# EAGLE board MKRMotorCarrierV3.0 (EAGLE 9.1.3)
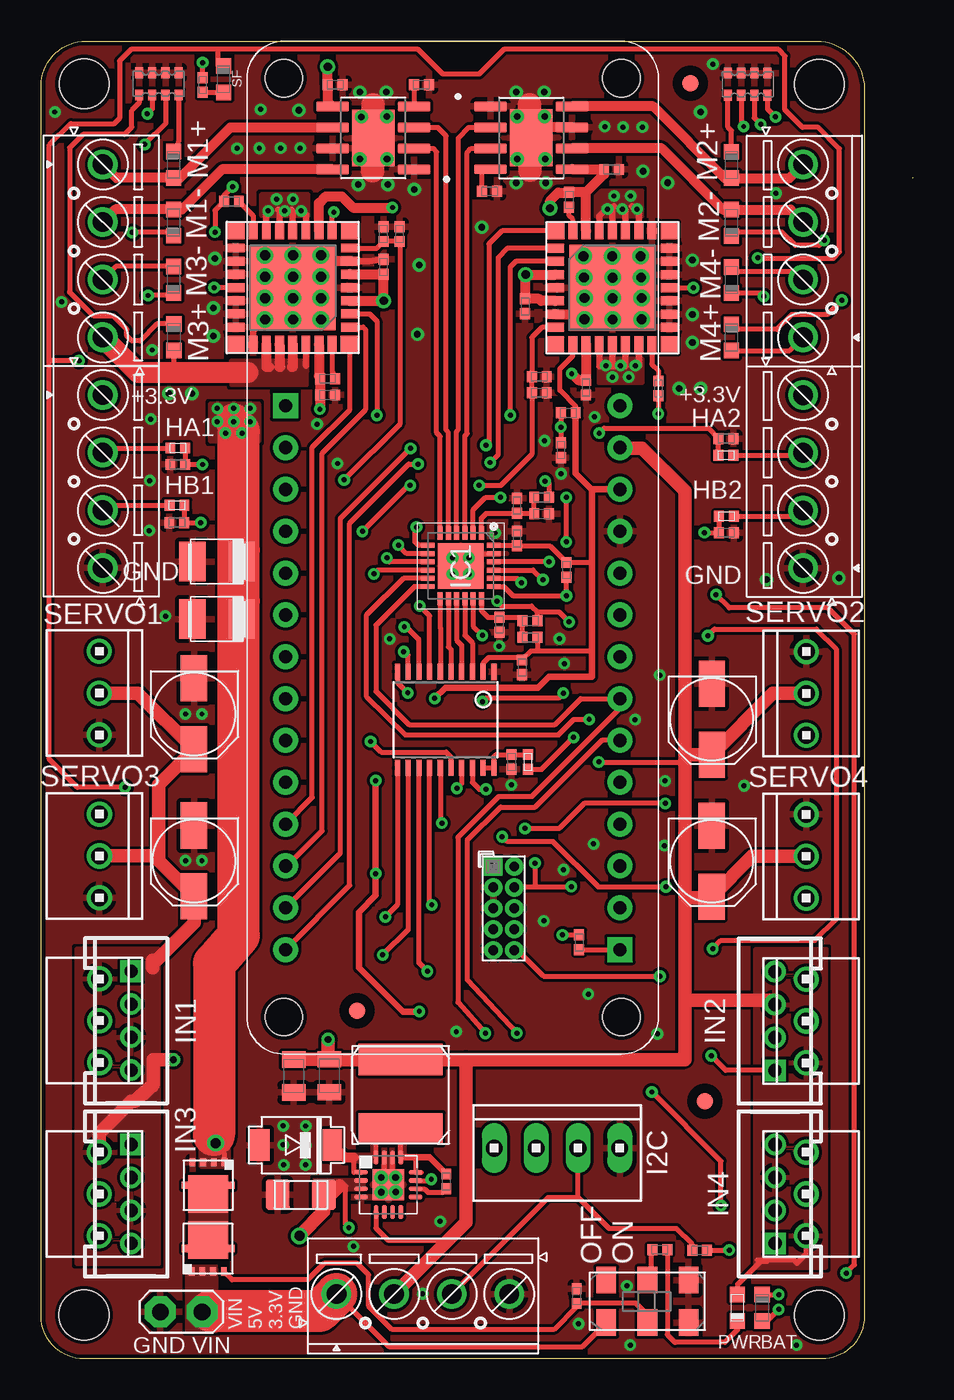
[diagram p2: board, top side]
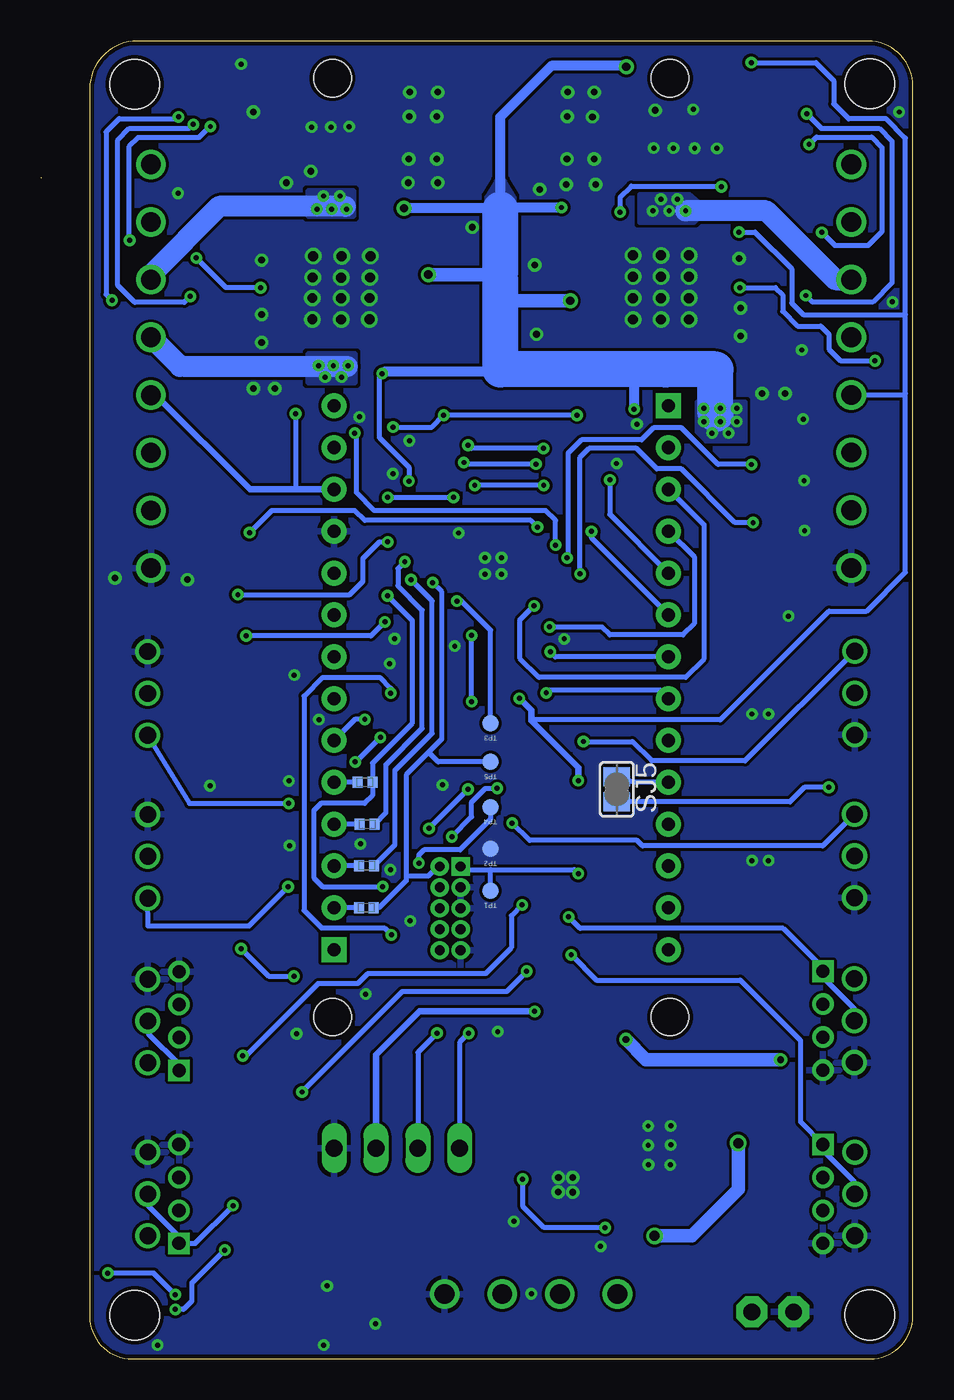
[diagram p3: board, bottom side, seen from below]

Size 52.95 x 80 mm. Coordinates in mm from the lower left corner, seen from the top.
Outline: 52.95,71.7 arc-90 52.95,71.7
Outline: 47.44,0 2.58,0 arc-90 0,2.58 0,77.28 arc-90 2.73,80 47.12,80 arc-90 50,77.12 50,2.56 arc-90 47.44,0
Copper layers (1*16): Top 0.035mm / dielectric 1.5mm / Bottom 0.035mm
Design rules "default *": minimum track width 0.3mm, minimum drill 0.3mm, track to track 7mil, track to pad 7mil, pad to pad 7mil, via to via 7mil, smd to smd 6mil, copper to edge 10mil, drill to drill 10mil, minimum pad ring 10mil, minimum via ring 8mil, stop-mask expansion 0.1mm, vias tented up to drill 0.5mm, thermal gap 10mil
Holes 3 mm at 2.6,2.66 47.26,2.64 47.27,77.39 2.61,77.41

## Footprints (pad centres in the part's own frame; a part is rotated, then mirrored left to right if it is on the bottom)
0402-1005X55N = smd 0.62 x 0.62: 1 -0.45,0; 2 0.45,0
SMC_B = smd 1.6 x 2.4: + -1.5,0; - 1.5,0
PANASONIC_C = smd 1.6 x 2.8: + 0,-2.15; - 0,2.15
C1206 = smd 1.8 x 1.45: 1 0,1.4; 2 0,-1.4
PINHEAD_2X05_127 = drill 0.6 pad 1.016 square: 1 -0.635,2.54 | drill 0.6 pad 1.016: 2 0.635,2.54; 3 -0.635,1.27; 4 0.635,1.27; 5 -0.635,0; 6 0.635,0; 7 -0.635,-1.27; 8 0.635,-1.27; 9 -0.635,-2.54; 10 0.635,-2.54
0805-R2013X50N = smd 0.95 x 1.45: 1 -1,0; 2 1,0
SOD-128 = smd 1.2 x 1.9: P$1 -2.2,0; P$2 2.2,0
LEDC1608X80N-AK = smd 0.9 x 0.95: A 0.8,0; C -0.8,0
QFN50P400X400X90-25N = smd 0.8 x 0.3: 1 -2,1.25; 2 -2,0.75; 3 -2,0.25; 4 -2,-0.25; 5 -2,-0.75; 6 -2,-1.25; 13 2,-1.25; 14 2,-0.75; 15 2,-0.25; 16 2,0.25; 17 2,0.75; 18 2,1.25 | smd 0.3 x 0.8: 7 -1.25,-2; 8 -0.75,-2; 9 -0.25,-2; 10 0.25,-2; 11 0.75,-2; 12 1.25,-2; 19 1.25,2; 20 0.75,2; 21 0.25,2; 22 -0.25,2; 23 -0.75,2; 24 -1.25,2 | smd 2.75 x 2.75: 25 0,0
MODULINO-3SM = drill 1.016: 1 2.54,0; 2 0,0; 3 -2.54,0
HW4-2.0 = drill 0.8 pad 1.27 square: 1 -3,0 | drill 0.8 pad 1.27: 2 -1,0; 3 1,0; 4 3,0
1X02 = drill 1.016 pad 1.88 octagon: 1 0,0; 2 2.54,0
6X6_NON-STANDARD = smd 1.9 x 5.1: P$1 -2.1,0; P$2 2.1,0
DFN3X3_8L = smd 0.5 x 0.35: P$1 -1.4,1.05; P$2 -1.4,0.4; P$3 -1.4,-0.25; P$4 -1.4,-0.9 | smd 2.28 x 2.45: P$5 0.51,0.055 | smd 0.43 x 0.38: P$6 0,1.47; P$7 0,-1.36
CAY16 = smd 0.5 x 0.65: 1 -1.2,-0.675; 2 -0.4,-0.675; 3 0.4,-0.675; 4 1.2,-0.675; 5 1.2,0.675; 6 0.4,0.675; 7 -0.4,0.675; 8 -1.2,0.675
SJ = smd 1.168 x 1.6: 1 -0.762,0; 2 0.762,0
TP-1.00MM = smd 1 x 1 bottom: X 0,0
MODULINO-4 = drill 1.016 long: 1 5.08,0; 2 2.54,0; 3 0,0; 4 -2.54,0
TSSOP20 = smd 0.305 x 0.991: 1 -2.925,-2.918; 2 -2.275,-2.918; 3 -1.625,-2.918; 4 -0.975,-2.918; 5 -0.325,-2.918; 6 0.325,-2.918; 7 0.975,-2.918; 8 1.625,-2.918; 9 2.275,-2.918; 10 2.925,-2.918; 11 2.925,2.918; 12 2.275,2.918; 13 1.625,2.918; 14 0.975,2.918; 15 0.325,2.918; 16 -0.325,2.918; 17 -0.975,2.918; 18 -1.625,2.918; 19 -2.275,2.918; 20 -2.925,2.918
QFN16 = smd 0.85 x 0.3: 1 -1.655,0.75; 2 -1.655,0.25; 3 -1.655,-0.25; 4 -1.655,-0.75; 9 1.655,-0.75; 10 1.655,-0.25; 11 1.655,0.25; 12 1.655,0.75 | smd 0.3 x 0.85: 5 -0.75,-1.655; 6 -0.25,-1.655; 7 0.25,-1.655; 8 0.75,-1.655; 13 0.75,1.655; 14 0.25,1.655; 15 -0.25,1.655; 16 -0.75,1.655 | smd 1.905 x 1.905: 17 0,0
32-PQFN(8X8) = smd 1.05 x 1.05: 1 -3.44,3.46; 9 -3.46,-3.46; 17 3.46,-3.46; 25 3.46,3.46 | smd 1.05 x 0.54: 2 -3.46,2.4; 3 -3.46,1.6; 4 -3.46,0.8; 5 -3.46,0; 6 -3.46,-0.8; 7 -3.46,-1.6; 8 -3.46,-2.4; 18 3.46,-2.4; 19 3.46,-1.6; 20 3.46,-0.8; 21 3.46,0; 22 3.46,0.8; 23 3.46,1.6; 24 3.46,2.4 | smd 0.54 x 1.05: 10 -2.4,-3.46; 11 -1.6,-3.46; 12 -0.8,-3.46; 13 0,-3.46; 14 0.8,-3.46; 15 1.6,-3.46; 16 2.4,-3.46; 26 2.4,3.46; 27 1.6,3.46; 28 0.8,3.46; 29 0,3.46; 30 -0.8,3.46; 31 -1.6,3.46; 32 -2.4,3.46 | smd 5.2 x 5.2: EPAD 0,0
SOIC127P600X170-8N = smd 1.97 x 0.6: 1 -2.475,1.905; 2 -2.475,0.635; 3 -2.475,-0.635; 4 -2.475,-1.905; 5 2.475,-1.905; 6 2.475,-0.635; 7 2.475,0.635; 8 2.475,1.905 | smd 2.58 x 3.45: 9 0,0
MKRBOARD-4CARRIER = drill 0.8 pad 1.524: 0 42.455,2.34; 1 44.995,2.34; 2 47.535,2.34; 3 50.075,2.34; 4 52.615,2.34; 5 55.155,2.34; 5V 22.135,22.66; 7 52.615,22.66; 8 50.075,22.66; 9 47.535,22.66; 10 44.995,22.66; 11 42.455,22.66; 12 39.915,22.66; 13 37.375,22.66; 14 34.835,22.66; A0 24.675,2.34; A1 27.215,2.34; A2 29.755,2.34; A3 32.295,2.34; A4 34.835,2.34; A5 37.375,2.34; A6 39.915,2.34; GND 29.755,22.66; RST 32.295,22.66; VCC 27.215,22.66; VIN 24.675,22.66 | drill 0.8 pad 1.524 square: 6 55.155,22.66; AREF 22.135,2.34 | hole 2.25: 59.25,2.25; 59.25,22.75; 2.25,22.75; 2.25,2.25
FD-1-1.5 = smd 1.016 x 1.016: P$1 0,0
CL-SB-22A = smd 1.2 x 1.6: P$1 -2.5,-1.29; P$2 0,-1.29; P$3 2.5,-1.29; P$4 -2.5,1.29; P$5 0,1.29; P$6 2.5,1.29
OSTTE/4 = drill 1.2: 1 -5.25,0; 2 -1.75,0; 3 1.75,0; 4 5.25,0

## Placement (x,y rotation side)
C1  100n  [0402-1005X55N]  28.9,49.81 90 top
C2  47uF  [SMC_B]  10.68,48.4 180 top
C3  47uF  [SMC_B]  10.68,44.91 180 top
C4  47n  [0402-1005X55N]  32.07,70.37 270 top
C5  150uF  [PANASONIC_C]  9.28,30.23 0 top
C6  47n  [0402-1005X55N]  17.4,59.51 0 top
C7  100n  [0402-1005X55N]  17.4,58.52 0 top
C8  100n  [0402-1005X55N]  34.65,72.21 0 top
C9  100n  [0402-1005X55N]  33.1,58.97 270 top
C10  1u  [0402-1005X55N]  21.77,68.29 270 top
C11  1u  [0402-1005X55N]  30.26,58.66 180 top
C12  100n  [0402-1005X55N]  29.4,63.9 270 top
C13  150uF  [PANASONIC_C]  40.73,30.21 0 top
C14  10n  [0402-1005X55N]  41.6,55.87 180 top
C15  10n  [0402-1005X55N]  41.62,50.15 0 top
C16  10n  [0402-1005X55N]  8.24,50.77 0 top
C17  10n  [0402-1005X55N]  8.3,54.3 180 top
C18  100n  [0402-1005X55N]  20.8,66.3 90 top
C19  100n  [0402-1005X55N]  28.58,36.24 270 top
C20  100n  [0402-1005X55N]  29.22,41.98 90 top
C21  100n  [0402-1005X55N]  28.9,51.8 90 top
C22  100n  [0402-1005X55N]  27.84,44.57 270 top
C23  10n  [0402-1005X55N]  32.53,3.81 270 top
C25  150uF  [PANASONIC_C]  9.28,39.16 0 top
C26  100n  [0402-1005X55N]  17.86,77.35 0 top
C31  150uF  [PANASONIC_C]  40.74,38.83 0 top
CBST  100n  [0402-1005X55N]  24.61,10.77 90 top
CBYPASS  10uF  [C1206]  15.77,9.97 90 top
CN1  DNP  [PINHEAD_2X05_127]  28.1,27.35 0 top
COUT1  22u  [0805-R2013X50N]  17.5,17.19 90 top
COUT2  22u  [0805-R2013X50N]  15.34,17.17 270 top
D1  40V/5A  [SOD-128]  15.49,12.98 180 top
DL1  YELLOW  [LEDC1608X80N-AK]  8.05,72.5 270 top
DL2  YELLOW  [LEDC1608X80N-AK]  8.05,68.99 90 top
DL3  YELLOW  [LEDC1608X80N-AK]  8.05,65.52 90 top
DL4  YELLOW  [LEDC1608X80N-AK]  8.06,62.03 270 top
DL5  YELLOW  [LEDC1608X80N-AK]  41.93,62.01 270 top
DL6  YELLOW  [LEDC1608X80N-AK]  41.93,65.5 90 top
DL7  YELLOW  [LEDC1608X80N-AK]  41.93,68.98 90 top
DL8  YELLOW  [LEDC1608X80N-AK]  41.93,72.49 270 top
DL9  ORANGE  [LEDC1608X80N-AK]  11.09,77.69 270 top
DL10  ORANGE  [LEDC1608X80N-AK]  43.8,3.1 270 top
FRAME1  DNP  [FRAME-NO-BAN]  not placed on the board
FRAME2  DNP  [FRAME]  not placed on the board
IC1  ATSAMD11D14A-MNT  [QFN50P400X400X90-25N]  25.49,48.14 270 top
IN1  DNP  [MODULINO-3SM]  3.55,20.53 90 top
IN2  DNP  [MODULINO-3SM]  46.47,20.51 270 top
IN3  DNP  [MODULINO-3SM]  3.53,10.01 90 top
IN4  DNP  [MODULINO-3SM]  46.47,10.01 270 top
J1  DNP  [HW4-2.0]  5.46,10.01 270 top
J2  DNP  [HW4-2.0]  5.46,20.53 270 top
J3  DNP  [HW4-2.0]  44.58,10.01 90 top
J4  DNP  [HW4-2.0]  44.57,20.51 90 top
JP2  M02PTH  [1X02]  7.24,2.85 0 top
LOUT  4.7uH/4A/35mO  [6X6_NON-STANDARD]  21.84,16.07 90 top
ON  GREEN  [LEDC1608X80N-AK]  42.3,3.1 90 top
Q1  AON7407  [DFN3X3_8L]  10.09,10.53 270 top
Q3  AON7407  [DFN3X3_8L]  10.2,6.7 90 top
R1  330R  [0402-1005X55N]  37.58,6.62 180 top
R2  39R  [0402-1005X55N]  29.7,44.8 0 top
R3  10k  [0402-1005X55N]  30.4,52.3 0 top
R4  140R  [0402-1005X55N]  41.6,54.86 0 top
R5  140R  [0402-1005X55N]  41.63,51.15 0 top
R6  140R  [0402-1005X55N]  8.25,51.83 180 top
R7  140R  [0402-1005X55N]  8.3,55.3 180 top
R8  DNP  [0402-1005X55N]  33.28,35 180 bottom
R9  3k3  [0402-1005X55N]  30.4,51.3 180 top
R10  200K  [0402-1005X55N]  29.57,36.24 270 top
R11  1k  [0402-1005X55N]  9.81,77.34 270 top
R12  10k  [0402-1005X55N]  32.02,57.43 0 top
R13  DNP  [0402-1005X55N]  33.15,32.46 180 bottom
R14  22K  [0402-1005X55N]  27.24,70.89 180 top
R15  DNP  [0402-1005X55N]  33.18,29.93 180 bottom
R16  DNP  [0402-1005X55N]  33.2,27.39 180 bottom
R17  22K  [0402-1005X55N]  23.1,77.35 180 top
R18  DNP  [0402-1005X55N]  31.57,55.17 90 top
R19  1k  [0402-1005X55N]  37.49,58.92 90 top
R20  1k  [0402-1005X55N]  11.56,70.27 0 top
R21  0R  [0402-1005X55N]  32.68,25.29 90 top
R22  270R  [0402-1005X55N]  30.26,59.62 180 top
R23  270R  [0402-1005X55N]  20.79,68.29 270 top
R24  330R  [0402-1005X55N]  40,6.6 0 top
R25  1k  [0402-1005X55N]  31.91,47.9 270 top
R26  10k  [0402-1005X55N]  29.7,43.8 180 top
RN2  1k  [CAY16]  42.92,77.39 180 top
RN4  1k  [CAY16]  7.15,77.41 180 top
SERVO1  DNP  [MODULINO-3SM]  3.53,40.42 90 top
SERVO2  DNP  [MODULINO-3SM]  46.48,40.4 270 top
SERVO3  DNP  [MODULINO-3SM]  3.54,30.53 90 top
SERVO4  DNP  [MODULINO-3SM]  46.47,30.51 270 top
SJ5  [SJ]  17.98,34.58 270 bottom
TP1  DNP  [TP-1.00MM]  25.64,28.42 180 top
TP2  DNP  [TP-1.00MM]  25.64,30.96 180 top
TP3  DNP  [TP-1.00MM]  25.64,38.58 180 top
TP4  DNP  [TP-1.00MM]  25.64,33.5 180 top
TP5  DNP  [TP-1.00MM]  25.64,36.24 180 top
TWI  -  [MODULINO-4]  32.61,12.79 180 top
U1  LSF0108  [TSSOP20]  24.57,38.8 180 top
U2  TS30013  [QFN16]  21.09,10.57 0 top
U3  MC33926PNB  [32-PQFN(8X8)]  15.28,65.04 180 top
U4  DRV8871  [SOIC127P600X170-8N]  20.18,74.12 180 top
U5  MC33926PNB  [32-PQFN(8X8)]  34.7,65.03 0 top
U7  DRV8871  [SOIC127P600X170-8N]  29.77,74.13 0 top
U$1  MKRBOARD4CARRIER  [MKRBOARD-4CARRIER]  12.5,80 270 top
U$33  DNP  [FD-1-1.5]  19.18,21.14 0 top
U$34  DNP  [FD-1-1.5]  40.32,15.63 0 top
U$35  DNP  [FD-1-1.5]  39.42,77.44 0 top
U$38  CL-SB-22A-02T  [CL-SB-22A]  36.83,3.49 180 top
X1  OSTTE/4  [OSTTE/4]  46.28,67.27 90 top
X2  OSTTE/4  [OSTTE/4]  46.28,53.26 90 top
X3  OSTTE/4  [OSTTE/4]  3.74,53.27 270 top
X6  OSTTE/4  [OSTTE/4]  3.74,67.27 270 top
X8  OSTTE/4  [OSTTE/4]  23.19,3.93 0 top

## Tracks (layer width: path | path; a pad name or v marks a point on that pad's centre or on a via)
+3.3V  (via drill 0.3)
  Top 0.305: U5.10 | U$1.VCC 35.15,52.8 | R11.1 v9.81,78.7 | R19.1 v37.49,57.38 | 30.1,42.99 29.78,42.99 C20.2 29.07,42.58 27.18,42.58 26.84,42.24 U1.2 | 30.1,42.99 33.47,42.99 | 32.61,9.8 TWI.3 | IC1.24 28.92,49.39 C1.1 30.91,49.36 R25.1 33.42,48.35 33.47,48.4 | U3.10 17.68,69.52 v17.78,69.62 | 32.61,9.8 34.51,7.9 38.6,7.9 39.55,6.95 R24.1 | X8.3 30.81,9.8 32.61,9.8 | 32.3,61.1 U5.10 | v10.56,68.41 10.56,69.72 R20.1 11.11,70.64 v11.63,71.16 | U5.10 32.3,60.9 31.5,60.1 31.5,58.8 32.47,57.83 R12.2 | R26.1 30.15,43.04 30.1,42.99
  Top 0.406: U$1.VCC 33.49,52.78 33.47,52.77 | v22.97,21.09 v22.96,21.08 21.97,21.08 19.3,23.75 19.3,27.12 20.32,28.14 v20.32,29.46 v20.32,35.11 | 33.47,52.77 33.47,48.4 33.47,42.99 33.47,41.4 30.84,41.4 30.19,40.75 24.55,40.75 v23.9,40.1 | R12.2 32.47,53.77 33.47,52.77
  Bottom 0.305: v9.81,78.7 5.89,78.7 4.8,77.61 4.8,76.19 3.89,75.28 1.61,75.28 0.45,74.12 0.45,63.4 | 0.45,58.6 0.45,47.75 2.8,45.4 5.1,45.4 11.7,38.8 23.1,38.8 23.16,38.73 | 0.45,58.6 0.45,63.4 | v37.49,57.38 37.49,52.78 | v17.78,69.62 17.78,70.52 17.1,71.2 11.67,71.2 v11.63,71.16 | 25.64,29.7 27.38,29.7 CN1.1 | 25.64,29.7 20.56,29.7 v20.32,29.46 | 0.45,63.4 6.66,63.4 7.35,64.09 7.35,66.17 9.59,68.41 v10.56,68.41 | TP1.X 25.64,29.7 | X3.1 0.53,58.52 0.45,58.6
  Bottom 0.406: U$1.VCC 37.49,52.78 40.26,52.78 45.98,58.51 X2.4 | v22.97,21.09 29.98,21.09 32.61,18.46 TWI.3 | v20.32,35.11 20.32,35.89 23.16,38.73 23.16,39.37 v23.9,40.1
+5V  (via drill 0.3, 0.4)
  Top 0.305: U2.5 20.34,7.93 21.07,7.2 24.71,7.2 25,7.5 | v33.87,36.24 33.89,36.22 39.07,36.22 39.1,36.25 | v32.34,37.73 30.4,35.79 R10.2 | IN4.1 46.47,6.37 45.9,5.8 45.7,6 43.5,6 43.6,5.9 44.1,5.9 44,6 43.8,6 42.3,4.5 ON.A
  Top 0.406: 39.11,18.18 39.1,18.17
  Top 0.813: LOUT.P$2 | LOUT.P$2 17.43,18.17 | 15.27,18.17 COUT2.1 15.36,18.19 COUT1.2 17.43,18.17 | LOUT.P$2 25.8,18.17 | 25.8,18.17 39.1,18.17 39.1,21.76 | 39.1,21.76 39.1,27.99 | 39.1,27.99 39.1,36.25 39.1,36.61 | 39.1,36.61 39.1,52.7 36.5,55.3 35.19,55.3 U$1.VIN | 39.1,36.61 39.17,36.68 C31.+ 44.46,40.4 SERVO2.2 | IN3.1 3.53,13.71 5.46,15.64 5.69,15.64 6.8,16.65 6.8,18.16 v8.04,18.16 | 6.77,24.21 6.77,23.96 | 6.77,23.96 6.77,23.73 | J4.3 44.52,21.76 39.1,21.76 | 39.1,27.99 40.66,27.99 C13.+ 43.18,30.51 SERVO4.2 | 7.13,30.23 C5.+ 9.28,26.47 6.77,23.96 | 7.13,30.23 7.13,34.86 C25.+ 5.87,40.42 SERVO1.2 | SERVO3.2 6.83,30.53 7.13,30.23 | 17.43,18.17 v17.43,19.39 | 25.8,18.17 25.8,8.29 25,7.5 X8.2
  Bottom 0.305: v33.87,36.24 33.83,36.24 v32.34,37.73
  Bottom 0.813: v8.04,18.16 16.2,18.16 v17.43,19.39
  pour Top: 7.13,24.88 2.16,24.88 2.16,5.8 7.14,5.8
  pour Top: 43.4,24.85 43.4,5.57 47.68,5.57 47.68,24.12 47.7,24.85
+VM  (via drill 0.3, 0.5, 0.5 pad 0.25, 0.6)
  Top 0.305: U4.5 | U3.31 16.93,61.58 | Q1.P$1 11.14,12.46 v10.6,13.1 | U2.11 23.62,10.82 v23.7,10.9 | R3.2 30.85,53.15 30.71,53.29 v30.61,53.29 | C2.+ 12.2,48.42 12,49.1 | C3.+ 12.2,44.93 12,46 | v18.69,7.96 18.5,8.15 18.5,10.5
  Top 0.61: U5.11 C9.1 32.63,59.42 v32.23,59.82 | U3.11 16.88,70.17 17.28,70.57 18.26,70.57 18.94,69.89 v21.33,69.89 v21.34,69.9 | v16.93,57.66 16.95,57.96 C7.1 C6.1 16.88,59.68 U3.31 | U5.31 33.1,70.82 | 33.1,70.82 C4.1 32.05,70.8 31.4,70.8 30.91,70.31 v30.91,69.86 | U7.5 34.2,72.22 C8.1 34.2,71.92 33.1,70.82 | U5.4 v29.43,65.83 29.4,65.8 C12.1 30.25,64.35 30.37,64.23 U5.6 | U3.4 v20.81,64.24 v20.8,64.25 C18.1 U3.6 | U4.5 17.41,76.32 C26.1 v17.41,78.45
  Top 0.813: CBYPASS.2 17.35,9.71 18.14,10.5 | 17.09,9.89 CBYPASS.2 | v15.69,7.47 17.17,8.95 CBYPASS.2
  Top 1.27: 10.5,13.6 10.5,13.2 v10.6,13.1
  Top 2.184: 12,56.3 v11.7,56.9
  Top 2.54: 12,56.3 12,49.1 12,46 12,25.7 10.5,24 10.5,13.6
  Bottom 0.305: v18.69,7.96 22.4,7.96 23.67,9.23 23.67,10.87 v23.7,10.9 | 25.27,59.92 25.06,59.92 25.06,60.07 | v30.61,53.29 30.61,54.14 32.4,55.93 32.4,59.65 v32.23,59.82
  Bottom 0.61: 25.06,69.78 25.06,69.86 | 25.06,69.86 v30.91,69.86 | v21.34,69.9 25.06,69.9 | 25.06,69.9 25.06,69.86 | 15,60.07 16.93,59.97 16.95,59.95 16.93,59.93 v16.93,57.66 | 25.27,59.92 32.13,59.92 v32.23,59.82 | 25.06,69.9 25.06,75.4 21.96,78.5 17.46,78.5 v17.41,78.45
  Bottom 0.813: v10.6,13.1 10.6,10.3 13.43,7.47 v15.69,7.47 | 24.9,65.84 25.06,66 | v29.43,65.83 25.39,65.83 25.06,65.5 | v20.81,64.24 25.06,64.24
  Bottom 1.27: 25.06,64.14 25.06,64.24
  Bottom 1.778: 25.06,65.5 25.06,66 | 25.06,64.1 25.06,64.24 25.06,64.4
  Bottom 2.184: 25.06,64.4 25.06,65.5 | 25.06,66 25.06,69.78 | 11.98,57.35 11.98,60.07 15,60.07 25.06,60.07 25.06,64.1
  other vias: 10.7,57.7 11.7,57.7 12.7,57.7 10.7,56.9 12.7,56.9 11.2,56.2 12.2,56.2
  pour Top (no thermals): 9.7,11.7 11.4,11.7 11.4,13.4 9.7,13.4
  pour Top: 13.2,55.7 10.3,55.7 10.3,58 13.2,58
  pour Bottom: 13.1,58.1 10.2,58.1 10.2,55.7 13.1,55.7
  pour Bottom: 24.2,69.9 24.2,70.5 24.8,71.5 25.3,71.5 25.9,70.5 25.9,69.9
  pour Top (no thermals): 19.61,10.85 16.57,10.85 17.8,10.3 19.6,10.3
/SF  (via drill 0.3)
  Top 0.305: U3.21 v10.51,65.04 | U5.21 v39.62,65.03 | DL9.C 10.75,78.53 10.75,79.5 | 10.75,79.5 5.46,79.5 4.76,78.8 4.76,75.32 4.44,75 1.8,75 0.5,73.7 0.5,60.6 | v5.1,34.7 2.2,34.7 0.5,36.4 0.5,60.6 | v2.3,60.6 0.5,60.6 | v43.53,66.84 43.47,66.8 48.1,66.8 48.5,67.2 48.5,73.47 47.2,74.77 46.25,74.77 45.19,75.83 45.19,79.11 44.8,79.5 28.1,79.5 26.6,78 24.4,78 22.9,79.5 10.75,79.5
  Bottom 0.305: SJ5.2 7.46,33.82 6.58,34.7 v5.1,34.7 | v39.62,65.03 41.72,65.03 v43.53,66.84 | v10.51,65.04 8.34,65.04 7.9,64.6 7.9,63.6 7,62.7 5.6,62.7 5.1,62.2 5.1,61.3 4.4,60.6 v2.3,60.6
A1  (via drill 0.3)
  Top 0.305: U1.7 23.59,45.12 v23,45.71
  Bottom 0.305: U$1.A1 12.67,50.62 12.67,42.51 13.81,41.37 22.7,41.37 23.88,42.55 23.88,44.83 v23,45.71
A2  (via drill 0.3)
  Top 0.305: U1.8 22.95,43.66 22.16,44.44 v22.06,44.44
  Bottom 0.305: U$1.A2 13.28,48.69 13.28,44.63 13.96,43.95 18.4,43.95 18.88,44.43 v22.05,44.43 v22.06,44.44
A5  (via drill 0.3)
  Top 0.305: U1.9 22.3,42.73 22.09,42.93 v22.02,42.93
  Bottom 0.305: 21.85,42.83 21.95,42.93 v22.02,42.93 21.71,42.62 U$1.A5
A6  (via drill 0.3)
  Top 0.305: U1.10 21.64,41.05 v22.27,40.43
  Bottom 0.305: U$1.A6 15.36,40.6 22.1,40.6 v22.27,40.43
FB_M3  (via drill 0.3)
  Top 0.305: v18.4,53.36 21.79,56.75 21.79,67.82 C10.2 R23.2 20.39,67.44 U3.8
  Bottom 0.305: v18.4,53.36 18.4,51.27 U$1.A3
FB_M4  (via drill 0.3)
  Top 0.305: v19.52,50.24 22.31,53.03 v22.42,53.03 | v26.61,53.03 27.93,53.03 29.81,54.91 C11.2 R22.2 29.81,62.01 30.43,62.63 U5.8
  Bottom 0.305: v22.42,53.03 v26.61,53.03 | U$1.A4 19.52,49.84 v19.52,50.24
GND  (via drill 0.3, 0.4, 0.41, 0.6)
  Top 0.305: U2.15 20.84,11.18 v20.66,11.01 | 21.33,12.2 21.33,11.21 v21.53,11.01 v21.52,11.01 | 25.09,48.95 IC1.25 25.79,48.14 26.54,48.89 IC1.23 | 33.14,64.33 33.13,64.33 v33.01,64.41 | 29.52,74.78 29.52,74.38 U7.9 | v32.98,65.65 34.71,65.05 v34.72,65.64 36.34,65.04 v36.45,65.65 | 33.14,63.03 33.13,63.03 v33.01,63.11
  Top 0.406: U3.7 19.89,66.64 C18.2 | U3.26 12.88,62.38 v13.6,63.1
  Top 0.61: U7.7 29.52,74.78 v28.92,75.43 | 33.14,64.33 33.18,64.29 33.18,64.41 U5.EPAD | 17.3,66.94 v17,67 17.36,66.64 U3.7 | U5.7 32.93,63.43 33,63.5 v33,64.4 v33.01,64.41 | 33.14,63.03 33.18,62.99 33.18,63.11 34.7,63.73 | v33,63.1 v33.01,63.11
  Top 1.422: 29.68,72.46 29.68,72.15 | 29.67,76.15 29.67,75.84 | 20.13,72.45 20.13,72.14 | 20.17,76.15 20.17,75.84
  other vias: 20.66,10.12 21.54,10.12 19.46,75.41 21.01,72.85 20.99,75.42 7.55,45.09 16.07,11.79 25.21,19.87 18.96,6.83 14.73,11.78 14.71,14.14 16.07,14.13 35.78,0.83 23.18,3.95 19.36,72.85 35.59,4.43 6.58,50.28 6.61,53.32 30.58,75.42 28.92,72.84 30.62,72.84 14.71,12.98 32.65,2.13 6.66,57.05 32.95,66.95 34.69,66.94 34.72,64.4 36.48,64.41 36.42,66.95 17,64.4 15.3,65.7 13.6,67 13.6,65.7 13.6,64.4 15.3,64.4 15.3,67 17,65.7 44.64,70.77 1.24,64.17 30.59,55.74 33.62,57.19 28.57,34.85 13.34,75.86 0.83,75.7 6.75,61.25 40.8,78.61 25.98,47.64 14.54,73.51 13.26,73.5 11.9,73.49 15.73,73.51 33.23,22.14 37.9,35.09 16.07,12.96 31.77,42.21 37.85,31.16 30.54,26.59 31.48,43.72 34.23,74.81 35.34,74.78 36.52,74.78 18,54.36 31.59,53.74 24.23,8.34 27.59,50.14 42.7,34.79 15.3,63.1 17,63.1 34.72,63.1 36.48,63.11 28.86,76.91 30.56,76.91 30.66,71.41 19.36,76.91 20.96,76.91 28.86,71.41 15.66,75.81 40.06,75.7 36.56,72.11 19.26,71.31 21.06,71.31 22.96,66.41 22.86,62.2 22.66,71 10.46,62.1 10.46,63.8 9.16,58.6 10.56,66.81 39.56,63.41 39.56,66.7 38.06,71.41 7.76,58.6 38.76,58.91 40.06,58.91 39.56,61.7 26.76,68.7 45.88,0.83 24.98,48.64 25.98,48.64 24.98,47.64 48.46,47.41 44.06,47.3 16.76,56.75 8.77,30.25 9.77,30.25 8.77,39.15 9.77,39.15 31.73,29.69 36.08,38.81 33.55,31.26 21.18,43.71 37.58,41.51 37.44,19.74 27.82,43.27
  pour Top (rank 6): 49.95,79.95 0.46,80.05 arc90 0.2,79.79 -0.13,-1.77 49.92,-1.77
  pour Bottom (rank 6): 0.05,79.8 -0.15,-1.79 48.01,-1.67 arc90 50.01,0.34 49.96,79.93
HA_E1  (via drill 0.3)
  Top 0.305: IC1.9 21.16,48.39 21,48.55 v21,48.63 | R7.1 C17.1 v9.8,54.3
  Bottom 0.305: v21,48.63 20.92,48.71 20.92,55 20.13,55.79 16.48,55.79 15.75,56.52 14.05,56.52 11.83,54.3 v9.8,54.3
HA_E2  (via drill 0.3)
  Top 0.305: R4.1 C14.2 40.52,56.5 34.2,56.5 v33.9,56.2 | IC1.8 22.21,48.89 v21.7,49.4
  Bottom 0.305: v21.7,49.4 21.7,50.9 22.3,51.5 32.7,51.5 33.8,52.6 33.8,56.1 v33.9,56.2
HB_E1  (via drill 0.3)
  Top 0.305: R6.1 C16.2 v9.7,50.77 | IC1.10 20.44,47.89 v20.21,47.66
  Bottom 0.305: v9.7,50.77 10.8,50.77 14.07,54.04 15.55,54.04 16.78,55.27 19.67,55.27 20.21,54.73 v20.21,47.66
HB_E2  (via drill 0.3)
  Top 0.305: R5.1 C15.1 v40.29,50.16 | IC1.7 22.91,49.39 22.7,49.6 22.7,50.4 v22.8,50.5
  Bottom 0.305: v22.8,50.5 23.2,50.9 33.3,50.9 33.9,51.5 38.95,51.5 v40.29,50.16
IN1_A6  (via drill 0.3)
  Top 0.305: U1.11 21.64,27.57 v20.91,26.83
  Bottom 0.305: IN1.2 3.55,21.25 5.46,23.16 J2.1 5.46,23.73 7.87,26.14 20.22,26.14 v20.91,26.83
IN1_M1
  Top 0.305: U4.3 24.09,74.75 24.6,74.25 24.6,56.39 24.74,56.25 IC1.5
IN1_M2
  Top 0.305: IC1.3 25.74,56.04 25.87,56.17 25.87,73.24 26.12,73.49 U7.3
IN1_M3
  Top 0.305: U3.2 19.56,62.64 19.7,62.5 19.7,57.61 17.07,54.98 17.07,32.05 14.94,29.93 U$1.3
IN1_M4  (via drill 0.3)
  Top 0.305: U5.2 28.34,67.43 27.77,66.86 27.77,54.92 v27.27,54.42 | U$1.5 18.74,28.75 18.74,50.73 22.33,54.32 v22.89,54.32
  Bottom 0.305: v22.89,54.32 27.17,54.32 v27.27,54.42
IN2_A1  (via drill 0.3)
  Top 0.305: U1.14 23.59,27.7 v23.73,27.56 | J4.1 41.59,17.51 v40.7,18.4
  Bottom 0.305: v23.73,27.56 24.38,26.91 24.38,24.97 25.96,23.39 33.11,23.39 33.7,22.8 36.1,22.8 40.5,18.4 v40.7,18.4 | IN2.2 46.47,19.77 44.57,17.87 J4.1
IN2_M1
  Top 0.305: IC1.6 24.24,56.01 24.03,56.22 24.03,73.27 23.82,73.48 U4.2
IN2_M2
  Top 0.305: IC1.4 25.24,56.32 25.34,56.42 25.34,74.12 25.99,74.77 U7.2
IN2_M3
  Top 0.305: U3.1 18.72,57.6 16.47,55.36 16.47,34.09 14.86,32.47 U$1.2
IN2_M4  (via drill 0.3)
  Top 0.305: U5.1 28,68.49 27.2,67.69 27.2,55.65 v27.02,55.47 v27.03,55.48 | v22.44,55.28 18.18,51.02 18.18,30.73 U$1.4
  Bottom 0.305: v22.44,55.28 26.83,55.28 v27.02,55.47
IN3_A5  (via drill 0.3)
  Top 0.305: U1.12 22.3,26.07 v20.75,24.52
  Bottom 0.305: v20.75,24.52 19.22,22.99 10.48,22.99 6.83,19.34 6.83,14.38 J1.1 5.46,12.65 3.53,10.72 IN3.2
IN4_A2  (via drill 0.3)
  Top 0.305: 22.96,35.87 U1.13 22.95,24.05 v23.46,23.53 | v41.3,9.3 41.3,12 v37.1,16.2
  Bottom 0.305: 31,22.31 30.99,22.31 | IN4.2 46.47,9.31 44.58,7.42 J3.1 43.59,7.01 v41.3,9.3 | v23.46,23.53 23.46,23.51 24.66,22.31 30.5,22.31 30.99,22.31 | v37.1,16.2 30.99,22.31
LED_S  (via drill 0.3)
  Top 0.305: IC1.2 26.24,51.54 27,52.3 v27.9,52.3 | DL10.C v44.8,3.9 | v41,46.4 41.8,45.6 47.8,45.6 49.4,44 49.4,5.7 v48.9,5.2 | v31.9,49.6 v31.9,52.3
  Bottom 0.305: v41,46.4 34.2,46.4 33.4,47.2 33.4,48.6 32.4,49.6 v31.9,49.6 | v31.9,52.3 v27.9,52.3 | v44.8,3.9 46.1,5.2 v48.9,5.2
M1+
  Top 0.61: U4.6 11.48,74.75 8.43,71.7 DL1.A 4.56,71.7 X6.1
M1-
  Top 0.61: U4.8 10.98,72.22 8.56,69.79 DL2.A 4.51,69.79 X6.2
M2+
  Top 0.61: U7.8 37.19,76.03 41.53,71.69 DL8.A 45.45,71.69 X1.4
M2-
  Top 0.61: U7.6 37.7,73.5 41.42,69.78 DL7.A 45.52,69.78 X1.3
M3+
  Top 0.305: DL4.A 8.06,59.91 8.04,59.89
  Top 0.406: U3.30 16.08,60.3
  Top 0.61: U3.29 15.28,60.22 15.23,60.22 | U3.28 14.48,60.22 14.52,60.22 | U3.27 13.68,60.22 13.87,60.22
  Top 1.27: 12.57,59.89 8.04,59.89 5.87,59.89 X6.4
  pour Top: 11.55,60.58 11.57,59.15 16.13,59.16 16.14,60.58
M3-  (via drill 0.3)
  Top 0.305: DL3.A 4.54,66.32 X6.3
  Top 0.406: U3.12 16.08,69.47 15.8,69.75 | U3.15 13.68,69.73 13.7,69.75 | U3.14 14.48,69.67 14.4,69.75 | U3.13 15.28,69.67 15.2,69.75
  Bottom 0.406: 15.97,69.75 15.95,69.75 15.88,69.67 15.82,69.67 v15.8,69.7
  Bottom 1.27: v13.8,69.7 8.9,69.7 4.72,65.52 X6.3
  other vias: 14.8,69.7 14.3,70.4 15.3,70.4
  pour Top (no thermals): 13.4,69.4 13.4,70.7 16.2,70.7 16.2,69.4
  pour Bottom: 13,70.2 13.6,70.7 16.6,70.7 16.6,69 13.3,69 13,69.3
M4+  (via drill 0.3)
  Top 0.305: DL5.A 45.47,61.21 X1.1
  Top 0.406: U5.12 33.9,60.26 34.34,60.25 | 34.7,60.26 34.71,60.26 | U5.13 34.7,60.26 | 34.7,60.26 34.34,60.25 | U5.14 35.5,60.26 34.34,60.25 | U5.15 36.3,60.26
  Bottom 1.27: 34.34,60.25 44.22,60.26 44.52,60.26 X1.1
  other vias: 34.3,60.3 35.2,60.3 36.1,60.3 35.7,59.6 34.7,59.6
  pour Top (no thermals): 33.87,60.7 33.87,59.29 36.51,59.29 36.51,60.7
  pour Bottom: 33.9,61 33.9,59.3 36.7,59.3 36.7,61
M4-  (via drill 0.3)
  Top 0.305: X1.2 45.8,66 41.93,66 DL6.A
  Top 0.406: U5.30 33.9,69.4 34.47,69.97 | U5.29 34.7,69.87 34.8,69.97 | U5.28 35.5,69.77 35.3,69.97 | U5.27 36.3,69.57 35.9,69.97
  Bottom 1.27: 34.47,69.97 42.13,69.97 46.28,65.82 X1.2
  other vias: 34.4,69.8 35.3,69.8 36.2,69.8 35.8,70.6 34.8,70.6
  pour Top (no thermals): 33.7,69.4 36.5,69.4 36.5,70.9 33.7,70.9
  pour Bottom: 34,69.4 36.7,69.4 36.7,70.9 34,70.9
MOSI  (via drill 0.3)
  Top 0.305: IC1.21 29.89,47.89 v30.48,47.3
  Bottom 0.305: R15.1 31.47,31.19 31.47,35.7 29.2,37.97 29.2,46.02 v30.48,47.3 30.48,47.18
N$2
  Top 0.305: R6.2 4.05,51.83 X3.3
N$3
  Top 0.305: U2.10 23.28,10.32 23.5,10.1 24.39,10.1 CBST.1 24.49,10.2
N$4  (via drill 0.3)
  Top 0.305: U1.16 24.89,36.53 24.6,36.83 20.66,36.83 v20.01,37.48
  Bottom 0.305: v20.01,37.48 17.04,37.48 15.86,36.3 10.19,36.3 SERVO1.1
N$5
  Top 0.305: 23.08,11.32 U2.12 22.75,12.22 | U2.1 19,11.32 19,12.22 | 20.34,13.97 LOUT.P$1 U2.13 22,12.22 | U2.16 20.34,13.6 20.8,13.6
  Top 0.406: 22,12.22 22.75,12.22 23.61,12.22 CBST.2
  Top 0.61: D1.P$1 18.45,12.22 19,12.22 | 19.8,13.6 20.8,13.6 21.84,13.6 LOUT.P$1
  pour Top (no thermals): 20.2,12.4 19,12.4 19,12 20.2,12
  pour Top (no thermals): 20.2,13.3 20.1,13.3 20.1,12.1 20.2,12.1
  pour Top (no thermals): 21.9,12.2 22.1,12.2 22.1,13.3 21.9,13.3
N$6  (via drill 0.3)
  Top 0.305: v37.95,28.66 33.84,28.66 31.1,31.4 28.3,31.4 v28,31.7 | U1.17 25.55,34.94 v25.25,34.64
  Bottom 0.305: v37.95,28.66 40.34,26.27 46.46,26.27 SERVO4.1 | v28,31.7 26.8,32.9 26.8,33.8 25.96,34.64 v25.25,34.64
N$7  (via drill 0.3)
  Top 0.305: U1.18 26.2,35.01 26.62,34.58 v27.02,34.58 | v37.91,33.72 33,33.72 31.48,32.2 v29.39,32.2
  Bottom 0.305: v37.91,33.72 43.93,33.72 SERVO2.1 | v29.39,32.2 v27.01,34.58 v27.02,34.58
N$9  (via drill 0.3)
  Top 0.305: U1.15 arc-90 U1.15 24.25,32.62 v24.34,32.53
  Bottom 0.305: SERVO3.1 5.47,31.14 16.42,31.14 16.75,31.47 23.28,31.47 v24.34,32.53
N$10
  Top 0.305: 7.82,55.32 R7.2 4.02,55.3 X3.2
N$11
  Top 0.305: R5.2 45.92,51.15 X2.2
N$12
  Top 0.305: R4.2 46.13,54.86 X2.3
N$13
  Top 0.305: R11.2 DL9.A
N$14  (via drill 0.3)
  Top 0.305: v37.59,23.23 30.52,23.23 28.93,24.81 CN1.10 | v40.5,43.9 40.9,44.3 47.1,44.3 48.3,43.1 48.3,26.7 47,25.4 41.3,25.4 v40.8,24.9 | 31.91,44.9 v32.07,44.74 31.46,45.35 30.15,45.35 | 30.15,45.35 29.8,45.7 28,45.7 v27.7,46 | R2.2 30.15,45.35
  Bottom 0.305: v32.07,44.74 32.91,43.9 v40.5,43.9 | v40.8,24.9 39.13,23.23 v37.59,23.23 | TP3.X 25.64,44.24 27.4,46 v27.7,46
N$15
  Top 0.305: IC1.18 26.74,45.43 27.15,45.02 C22.1 29.03,45.02 R2.1 R26.2
N$16
  Bottom 0.305: U$1.1 16.96,35.01 SJ5.1
N$17
  Top 0.305: RN4.8 8.35,73.9 DL1.C
N$18
  Top 0.305: U1.19 U1.20 27.5,36.55 27.63,36.69 C19.1 R10.1
N$19
  Top 0.305: 37.04,4.69 U$38.P$2 | U$38.P$2 36.65,4.68 | R1.2 37.03,6.52 37.03,4.98 U$38.P$2
N$20  (via drill 0.3)
  Top 0.305: v6.3,73.73 7.55,74.98 RN4.7 | DL2.C 7.85,68.39 v5.53,68.39
  Bottom 0.305: v6.3,73.73 5.86,74.17 2.5,74.17 1.87,73.54 1.87,68.43 2.7,67.6 4.74,67.6 v5.53,68.39
N$21  (via drill 0.3)
  Top 0.305: RN4.6 6.75,75.89 v6.45,75.59 | DL3.C 7.89,64.56 v6.5,64.56
  Bottom 0.305: v6.45,75.59 5.56,74.7 2.04,74.7 1.27,73.93 1.27,65.33 2.44,64.16 6.1,64.16 v6.5,64.56
N$22
  Top 0.305: Q1.P$7 9.63,10.53 Q1.P$5 Q1.P$6 | Q3.P$6 Q3.P$5 Q3.P$7
  pour Top (no thermals): 11.06,10.8 9.23,10.8 9.23,7.2 11.07,7.21
N$23
  Top 0.305: 32.72,3.37 C23.2 | C23.2 arc-90 32.77,3.4 36.1,3.4 36.7,2.8 36.7,2.33 U$38.P$5 | Q3.P$4 11.6,4.8 16.2,4.8 17.2,5.8 19.2,5.8 19.9,5.1 19.9,3.2 21.33,1.77 31.14,1.77 32.53,3.16 C23.2
N$24  (via drill 0.3)
  Top 0.305: RN2.8 44.12,75.89 v44.61,75.4 | v48.64,64.27 47.77,63.4 45.6,63.4 44.7,62.5 42.24,62.5 DL5.C
  Bottom 0.305: v48.64,64.27 49,64.63 49,74.5 48.2,75.3 44.71,75.3 v44.61,75.4
N$25
  Top 0.305: RN4.5 5.95,76.25 5.5,75.8 5.5,74.78 5.06,74.34 2.54,74.34 1.73,73.53 1.73,64.77 3.2,63.3 4.4,63.3 5.2,62.5 5.2,62.1 5.5,61.8 6,61.8 7.03,62.83 DL4.C
N$26  (via drill 0.3)
  Top 0.305: RN2.7 43.32,75.34 v43.71,74.95 | v43.89,64.5 43.69,64.7 DL6.C
  Bottom 0.305: v43.71,74.95 43.96,74.7 47.6,74.7 48.3,74 48.3,65.18 47.26,64.14 44.25,64.14 v43.89,64.5
N$28
  Top 0.305: U3.32 17.68,59.98 C6.2
N$30
  Top 0.305: U5.32 32.3,69.18 32.07,69.41 C4.2
N$31  (via drill 0.3)
  Top 0.305: 41.92,68.32 DL7.C 42.15,68.4 45,68.4 45.8,67.6 47.26,67.6 v47.57,67.91 | 42.72,74.87 v42.67,74.82 42.52,74.97 RN2.6
  Bottom 0.305: v42.67,74.82 43.39,74.14 47.06,74.14 47.62,73.58 47.62,68.26 v47.57,67.91
N$32
  Top 0.305: DL8.C 41.93,74.57 41.72,74.78 RN2.5
N$35
  Top 0.305: U3.16 12.88,69.4 R20.2
N$36
  Top 0.305: R17.2 U4.4
N$37
  Top 0.305: U5.16 37.1,60.4 37.49,60.01 R19.2
N$38
  Top 0.305: R21.1 U$1.6
N$39
  Top 0.305: U7.4 26.79,72.22 R14.2
  Top 0.406: 27.22,72.23 U7.4 27.22,72.24
N$40
  Bottom 0.305: R8.2 U$1.10
N$41
  Bottom 0.305: U$1.9 R13.2
N$42  (via drill 0.3)
  Top 0.305: R24.2 v41.8,6.6 | v44.8,3 44.1,2.3 DL10.A
  Bottom 0.305: v44.8,3 44.3,3 43.8,3.5 43.8,4.6 v41.8,6.6
N$43
  Bottom 0.305: R15.2 U$1.8
N$45
  Bottom 0.305: R16.2 U$1.7
N$133
  Top 0.305: 42.6,2.06 ON.C 42.3,1.76 41.54,1 38.5,1 38.03,1.47 R1.1
PWRIN
  Top 0.305: 33.9,2.2 U$38.P$6 32.87,0.74 21.13,0.74 X8.1
  Top 1.778: 9.97,3.04 JP2.2
  Top 2.54: X8.1 16.91,2.9 10.3,2.9
  pour Top (no thermals): 8.9,5.6 10.6,5.6 10.6,1.7 8.9,1.7
SCK  (via drill 0.3)
  Top 0.305: v30.86,48.39 IC1.22
  Bottom 0.305: R13.1 32.02,33.14 32.02,36.05 29.8,38.27 29.8,45.46 31.28,46.94 31.28,47.97 v30.86,48.39
SCL  (via drill 0.3)
  Top 0.305: IC1.12 22.68,46.89 20.33,44.54 20.33,40.53 22.36,38.5 31.2,38.5 32.78,40.09 U$1.12 35.16,39.49 29.82,34.15 27.8,34.15 25.31,31.66 25.31,21.64 v26.98,19.77
  Bottom 0.305: v26.98,19.77 27.53,19.22 TWI.1
SD11_INT  (via drill 0.3)
  Top 0.305: IC1.17 26.24,44.48 v26.8,43.92 | v31.67,25.74 R21.2 | v26.8,39.9 27.02,40.12 31.42,40.12 v31.72,40.42
  Bottom 0.305: v26.8,39.9 v26.8,43.92 | v31.67,25.74 32.1,26.17 35.92,26.17 36.98,27.23 36.98,40.24 35.85,41.37 32.37,41.37 31.72,40.72 v31.72,40.42
SDA  (via drill 0.3)
  Top 0.305: IC1.11 22.02,47.39 19.77,45.19 19.77,40.19 22.12,37.89 31.43,37.89 32.36,38.82 v33.29,38.82 | U$1.11 34.05,37.55 30.01,33.5 27.91,33.5 25.88,31.47 25.88,23 v28.9,19.78
  Bottom 0.305: U$1.11 33.88,38.82 v33.29,38.82 | v28.9,19.78 30.07,18.61 TWI.2
SERVO1
  Top 0.305: IC1.14 24.74,43.22 24.9,43.06 U1.5
SERVO2
  Top 0.305: IC1.16 25.74,43.92 26.19,43.47 U1.3
SERVO3
  Top 0.305: IC1.13 24.24,44.39 24.25,44.38 U1.6
SERVO4
  Top 0.305: IC1.15 25.24,43.64 25.55,43.34 U1.4
SLEW  (via drill 0.3)
  Top 0.305: 31.57,55.69 R18.2 v31.57,56.57 R12.1 | U5.3 28.83,66.63 28.48,66.28 28.48,57.41 28.5,57.39 v28.5,57.29 | v20.4,57.29 20.4,63 19.96,63.44 U3.3
  Bottom 0.305: v20.4,57.29 v28.5,57.29 29.22,56.57 v31.57,56.57
SWCLK/MISO  (via drill 0.3)
  Top 0.305: v31.91,46.33 28.66,46.33 28.1,46.89 IC1.19 | v31.91,46.33 v31.9,46.34 | CN1.4 28.89,28.67 30,28.67 | 30,28.67 v32.2,28.67 | v30,30.1 30,28.67 | v31.91,46.33 R25.2
  Bottom 0.305: v32.2,28.67 35.86,28.67 36.4,29.21 36.4,33.29 35.96,33.73 33.3,33.73 32.83,34.2 R8.1 32.83,36.17 30.4,38.6 30.4,44.82 v31.91,46.33 31.73,46.33 | TP4.X 25.64,32.76 27.5,30.9 29.7,30.9 30,30.6 v30,30.1
SWDIO/SS  (via drill 0.3)
  Top 0.305: IC1.20 28.91,47.39 v29.17,47.13
  Bottom 0.305: 29.42,36.82 30.78,35.46 30.78,29.3 | 30.78,29.3 30.78,29.02 32.41,27.39 R16.1 | TP5.X 28.84,36.24 29.42,36.82 | 29.42,36.82 28.6,37.64 28.6,46.56 v29.17,47.13 | 30.78,29.3 29.45,29.3 28.84,29.9 28.84,29.89 CN1.2
V_READ
  Top 0.305: IC1.1 26.74,51.04 27.01,51.31 R9.2 | R9.2 R3.1 | R9.2 28.9,51.3 C21.1

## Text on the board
tPlace: PWR | BAT
tNames: SF | M1+ | M2+ | M1- | M3- | M2- | M3+ | M4- | M4+ | +3.3V | +3.3V | HA2 | HA1 | HB1 | HB2 | GND | GND | I2C | OFF / ON | VIN / 5V / 3.3V / GND | GND VIN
